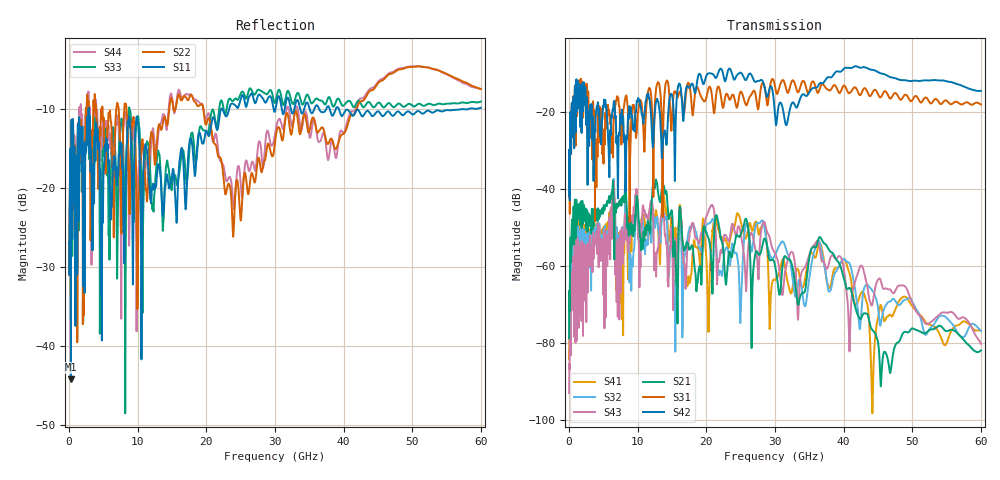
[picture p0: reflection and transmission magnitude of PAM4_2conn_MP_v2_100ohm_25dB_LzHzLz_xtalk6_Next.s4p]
! Info: Touchstone file created by Circ.  Input file=FAB50GbE_2conn_Midplane_Examax_Topo2_v2_100ohm_25dB_LzHzLz.circ
# Hz S RI R 50
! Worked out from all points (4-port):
!   6000 points, 10 MHz to 60 GHz, reference 50 ohm
!   strongest paths, dB at 10 MHz, 15.01 GHz, 30.01 GHz, 45.01 GHz, 60 GHz:
!     S42: -41.8, -15.8, -21.2, -9.7, -14.6
!     S31: -42.1, -21.7, -13.4, -15.4, -18.1
!     S21: -78.8, -46.1, -59.9, -79.8, -82.0
!     S43: -93.1, -52.6, -56.7, -63.6, -80.2
!     S32: -78.4, -52.4, -57.3, -70.9, -76.9
!     S41: -84.4, -48.0, -63.8, -73.5, -76.9
!   lowest |S11| = -44.2 dB at 270 MHz (marker M1), VSWR 1.01, Z = 49.6 + j0.445 ohm
!   |S11| at or under -10 dB: start of sweep to 2.828 GHz; 2.862 GHz to 22.14 GHz (19.27 GHz wide, 154 % of centre); 39.33 GHz to 56.93 GHz (17.6 GHz wide, 36.6 % of centre)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
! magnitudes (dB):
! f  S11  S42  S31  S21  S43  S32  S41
! 10 MHz  -30.9  -41.8  -42.1  -78.8  -93.1  -78.4  -84.4
! 270 MHz  -44.2  -25.6  -25.6  -56.0  -76.6  -62.1  -64.5
! 6.38 GHz  -17.6  -19.7  -31.1  -38.3  -43.0  -40.6  -42.4
! 12.55 GHz  -19.8  -19.3  -16.5  -39.0  -57.5  -49.8  -47.8
! 15.51 GHz  -21.7  -24.5  -14.8  -57.4  -53.5  -73.9  -50.2
! 20.77 GHz  -11.6  -10.1  -15.2  -60.6  -44.2  -48.3  -53.2
! 60 GHz  -9.8  -14.6  -18.1  -82.0  -80.2  -76.9  -76.9
